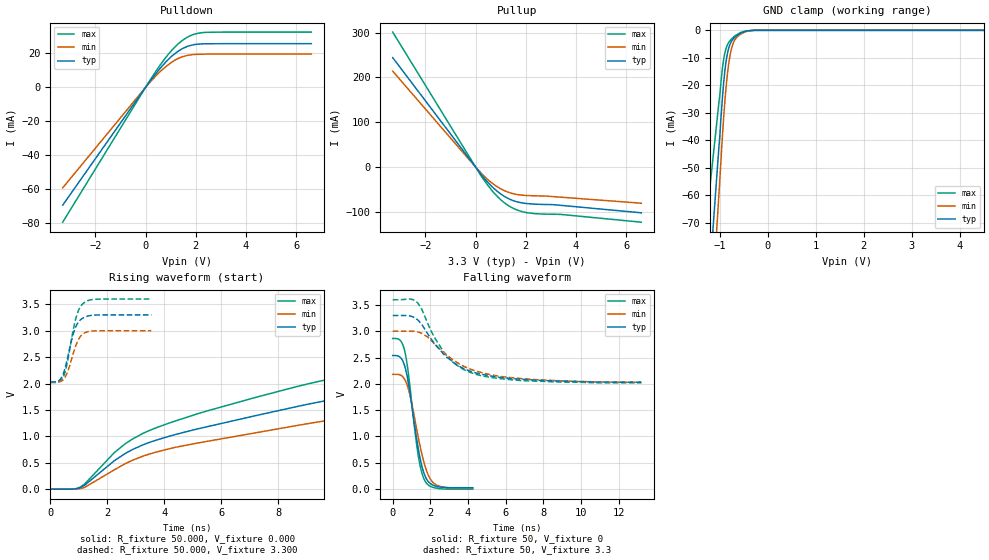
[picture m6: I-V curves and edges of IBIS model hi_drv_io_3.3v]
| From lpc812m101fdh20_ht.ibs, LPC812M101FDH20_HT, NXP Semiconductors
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[Model]   hi_drv_io_3.3v
Model_type I/O
Vinl=9.900E-01
Vinh=2.310E+00
Vref=0.000E+00
Rref=1.000E+06
Cref=2.000E-11
Vmeas=1.650E+00
C_comp   8.440E-13   8.280E-13   8.600E-13
[Voltage Range]   3.300E+00   3.000E+00   3.600E+00
[POWER Clamp Reference]   3.300E+00   3.000E+00   3.600E+00
[GND Clamp Reference]   0.000E+00   0.000E+00   0.000E+00
[Pullup Reference]   3.300E+00   3.000E+00   3.600E+00
[Pulldown Reference]   0.000E+00   0.000E+00   0.000E+00
[Temperature Range]   25   105   -40
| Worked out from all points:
|   slope of the pulldown table from 0 to 0.495 V, typ, clamps not added: 51.2 ohm
|   slope of the pullup table from 0 to 0.495 V, typ, clamps not added: 14.4 ohm
|   GND clamp passes 1 mA (typ) near -0.56 V on its own axis
|   rising waveform, R_fixture 50.000, V_fixture 0.000: 20-80 % time 11.3ns typ, 13ns min, 9.8ns max; typ from 0 V to 2.52 V
|   falling waveform, R_fixture 50, V_fixture 0: 20-80 % time 666ps typ, 760ps min, 590ps max; typ from 2.54 V to 0.022 V
|   rising waveform, R_fixture 50.000, V_fixture 3.300: 20-80 % time 360ps typ, 355ps min, 352ps max; typ from 2.03 V to 3.3 V
|   falling waveform, R_fixture 50, V_fixture 3.3: 20-80 % time 2.11ns typ, 2.53ns min, 1.78ns max; typ from 3.3 V to 2.03 V
[GND Clamp]
-3.3V     -590.4mA   -705.8mA   -398.8mA
-1.02V    -42.46mA   -59.51mA   -26.24mA
-1V       -38.06mA   -54.12mA   -23.49mA
-960mV    -27.61mA   -42.2mA    -15.89mA
-920mV    -18.88mA   -31.48mA   -10.45mA
-880mV    -12.49mA   -22.47mA   -7.085mA
-820mV    -6.778mA   -12.65mA   -4.527mA
-780mV    -4.748mA   -8.414mA   -3.589mA
-720mV    -3.081mA   -4.622mA   -2.525mA
-560mV    -993.4uA   -1.291mA   -739uA
-280mV    0A         0A         0A
6.6V      0A         0A         0A
[POWER Clamp]
-3.3V     0A         0A         0A
6.6V      0A         0A         0A
[Pullup]
-3.3V     244.2mA    214mA      301.2mA
200mV     -14.86mA   -12.04mA   -18.13mA
440mV     -31.15mA   -25.75mA   -37.26mA
700mV     -46.18mA   -37.64mA   -55.7mA
1.14V     -65.29mA   -52.43mA   -79.52mA
1.56V     -76.12mA   -60.21mA   -93.77mA
2.1V      -81.83mA   -63.74mA   -102.3mA
3.38V     -85.45mA   -67.25mA   -105.8mA
6.6V      -102.2mA   -80.79mA   -123.1mA
[Pulldown]
-3.3V     -69.61mA   -59.39mA   -79.67mA
160mV     3.297mA    2.77mA     3.818mA
560mV     10.84mA    8.974mA    12.7mA
900mV     16.39mA    13.31mA    19.41mA
1.16V     19.76mA    15.97mA    23.66mA
1.44V     22.62mA    17.89mA    27.44mA
1.66V     24.17mA    18.82mA    29.56mA
1.88V     25.03mA    19.33mA    31.09mA
2.4V      25.7mA     19.6mA     32.46mA
6.6V      25.77mA    19.62mA    32.62mA
[Rising Waveform]
R_fixture = 50.000
V_fixture = 0.000
V_fixture_min = 0.000
V_fixture_max = 0.000
|  time   V(typ)   V(min)   V(max)
0s        0V         0V         0V
1.05ns    29.02mV    10.41mV    37.02mV
2.6ns     664.8mV    473.1mV    846.3mV
4.1ns     990.2mV    755.5mV    1.237V
8.7ns     1.569V     1.209V     1.949V
12.8ns    1.963V     1.549V     2.383V
16.1ns    2.184V     1.761V     2.593V
20.6ns    2.352V     1.956V     2.73V
26.8ns    2.457V     2.087V     2.819V
34.5ns    2.517V     2.16V      2.872V
[Falling Waveform]
R_fixture = 50
V_fixture = 0
V_fixture_min = 0
V_fixture_max = 0
0s        2.538V     2.18V      2.862V
400ps     2.504V     2.168V     2.826V
650ps     2.324V     2.076V     2.604V
950ps     1.745V     1.732V     1.836V
1.35ns    780.9mV    991.5mV    650.4mV
1.5ns     506.7mV    734.7mV    369.5mV
1.7ns     260.1mV    451.7mV    160mV
2ns       101.3mV    185.2mV    48.52mV
2.35ns    46.32mV    69.21mV    12.63mV
4.25ns    21.97mV    19.54mV    -5.31mV
[Rising Waveform]
R_fixture = 50.000
V_fixture = 3.300
V_fixture_min = 3.000
V_fixture_max = 3.600
|  time   V(typ)   V(min)   V(max)
0s        2.03V      2.028V     2.019V
300ps     2.055V     2.031V     2.031V
450ps     2.176V     2.069V     2.115V
600ps     2.47V      2.209V     2.402V
750ps     2.827V     2.466V     2.854V
850ps     3.013V     2.647V     3.13V
1ns       3.172V     2.845V     3.397V
1.15ns    3.241V     2.941V     3.515V
1.55ns    3.296V     2.997V     3.595V
3.55ns    3.3V       3V         3.6V
[Falling Waveform]
R_fixture = 50
V_fixture = 3.3
V_fixture_min = 3
V_fixture_max = 3.6
0s        3.3V       3V         3.6V
950ps     3.288V     3V         3.611V
1.3ns     3.224V     2.989V     3.548V
1.55ns    3.127V     2.959V     3.415V
2.2ns     2.774V     2.765V     2.896V
2.75ns    2.548V     2.581V     2.589V
3.45ns    2.351V     2.397V     2.342V
4.25ns    2.224V     2.262V     2.2V
7.4ns     2.074V     2.083V     2.053V
13.2ns    2.03V      2.028V     2.019V
[Ramp]
dV/dt_r   1.5096E+00/1.1289E-08   1.2961E+00/1.3054E-08   1.7205E+00/9.8063E-09
dV/dt_f   7.6204E-01/2.1066E-09   5.8333E-01/2.5229E-09   9.4867E-01/1.7695E-09
R_load = 50
